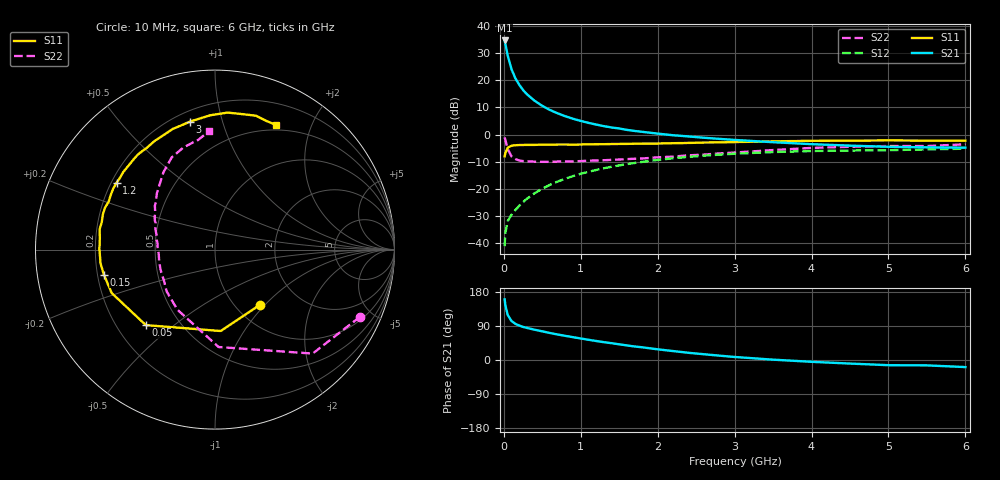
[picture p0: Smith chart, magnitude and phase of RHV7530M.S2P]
! SIEMENS Small Signal Semiconductors
! BFR106
! Si NPN RF Bipolar Junction Transistor in SOT23
! VCE = 0.75 V  IC = 30 mA
! Common Emitter S-Parameters:  August  1996
# GHz  S  MA  R  50
!  f  S11  S21  S12  S22
! GHz  MAG  ANG  MAG  ANG  MAG  ANG  MAG  ANG
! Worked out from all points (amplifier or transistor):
!   36 points, 10 MHz to 6 GHz, reference 50 ohm
!   highest |S21| = 34.5 dB at 10 MHz (marker M1)
!   |S21| within 3 dB of that: start of sweep to 32.22 MHz
!   unconditionally stable (mu >= 1): 256.2 MHz to end of sweep
!   at 250 MHz: K = 0.99, MSG = 20.6 dB, |S12| = -24.8 dB
!   at 1.4 GHz: K = 1.09, MAG = 5.4 dB, |S12| = -11.8 dB
!   at 6 GHz: K = 1.03, MAG = -0.8 dB, |S12| = -5.2 dB
!   S11 on the Smith chart (normalised r, x): 10 MHz: 1.28, -0.94; 50 MHz: 0.32, -0.40; 150 MHz: 0.23, -0.11; 1.2 GHz: 0.22, +0.29; 3 GHz: 0.26, +0.79; 6 GHz: 0.44, +1.51
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0.01  0.3965 -51.2  53.38 160.1  0.0089 75.5  0.8903 -24.9
0.02  0.4547 -86.0  46.24 144.6  0.0157 64.0  0.7947 -46.8
0.05  0.5706 -132.5  28.18 118.7  0.0256 49.6  0.5431 -87.9
0.1  0.6245 -157.2  15.81 102.9  0.0338 48.9  0.3949 -122.1
0.15  0.6346 -167.3  10.76 95.5  0.0412 53.8  0.3559 -139.3
0.2  0.6424 -173.1  8.191 90.9  0.049 57.5  0.3321 -149.1
0.25  0.6421 -177.3  6.551 87.3  0.0574 59.8  0.3255 -156.8
0.3  0.6441 179.8  5.488 84.7  0.0661 62.2  0.3219 -161.3
0.4  0.6448 174.3  4.165 79.9  0.0835 63.9  0.3174 -168.6
0.5  0.6527 170.0  3.353 75.6  0.1009 64.8  0.3149 -173.6
0.6  0.6491 166.4  2.818 71.3  0.1194 64.6  0.3149 -176.9
0.7  0.655 162.4  2.445 67.3  0.137 64.0  0.3185 180.0
0.9  0.6498 155.8  1.946 60.2  0.1727 61.6  0.3213 174.2
1.1  0.6611 149.0  1.638 53.3  0.2067 58.8  0.3307 170.2
1.2  0.6631 145.8  1.524 50.2  0.2232 57.2  0.3338 167.9
1.7  0.6773 131.9  1.163 35.7  0.3001 48.5  0.359 157.7
2.2  0.6926 119.0  0.97 23.6  0.3656 39.6  0.393 148.0
3  0.7267 101.0  0.796 8.0  0.4433 25.7  0.4663 132.4
3.5  0.7484 92.2  0.722 0.9  0.4763 18.1  0.518 123.7
4.5  0.7701 78.5  0.625 -9.4  0.5075 4.4  0.5951 107.3
5.5  0.7718 67.8  0.581 -14.2  0.5328 -3.8  0.6137 99.5
6  0.7729 64.0  0.574 -18.7  0.549 -10.0  0.6614 92.7
